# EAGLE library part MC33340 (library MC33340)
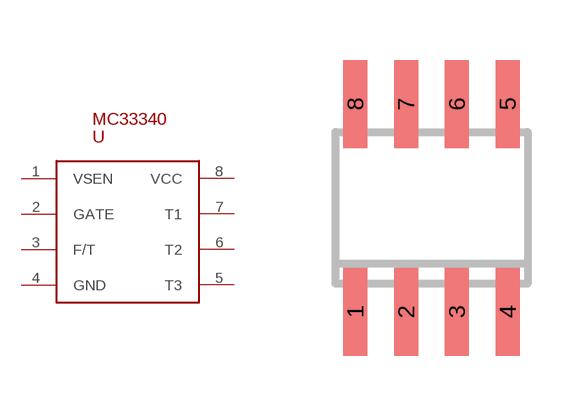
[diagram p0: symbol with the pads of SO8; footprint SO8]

Designator prefix -

## MC33340  [SO8]
1  VSEN
2  GATE
3  F/T
4  GND
5  T3
6  T2
7  T1
8  VCC

## Footprint SO8 (pad centres in mm)
SMALL OUTLINE INTEGRATED CIRCUIT
smd 0.6 x 2.2: 1 -1.905,-2.6; 2 -0.635,-2.6; 3 0.635,-2.6; 4 1.905,-2.6; 5 1.905,2.6; 6 0.635,2.6; 7 -0.635,2.6; 8 -1.905,2.6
